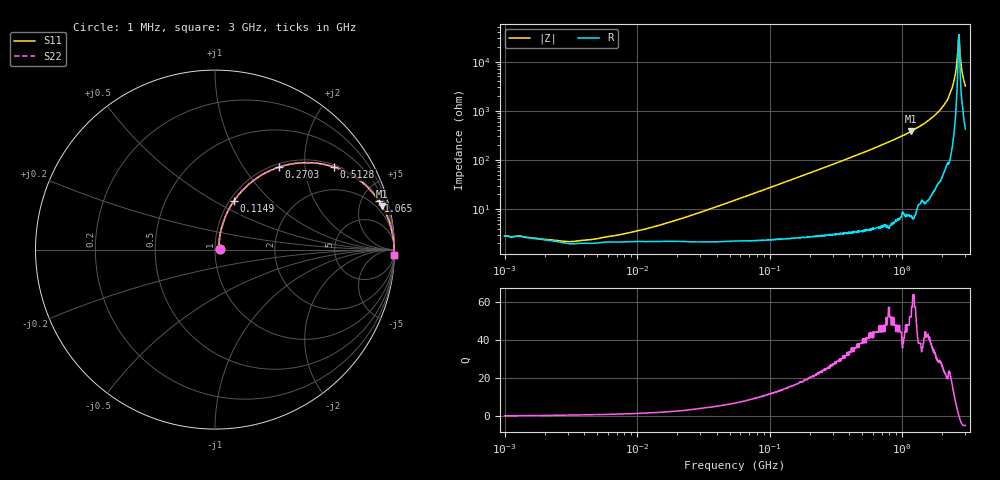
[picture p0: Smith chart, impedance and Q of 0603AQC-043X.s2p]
!s-Parameter Generated by FASTRON Sdn. Bhd.
!FASTRON P/N : 0603AQC-043X
!Keysight Technologies: E4991B_MY54100416_A.01.15
!Date: Thu Jun 25 13:54:13 2026
!Version  :Rev00  Thu Jun 25 13:54:13 2026
!Data & Calibration Information:
!Freq  S11  S21  S12  S22
!PortZ  Port1:50+j0  Port2:50+j0
!When reading reference impedance value at option line is always used.
! Remarks : This data is being provided solely for informational purposes.
# Hz S dB R 50
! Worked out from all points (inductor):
!   1601 points, 1 MHz to 3 GHz, reference 50 ohm
!   read as one part in series: L = 44 nH near 23.51 MHz
!   highest Q = 52.2 at 1.171 GHz (marker M1), where L = 52.1 nH
!   self-resonance near 2.674 GHz
!   S11 on the Smith chart (normalised r, x): 1 MHz: 1.06, +0.01; 114.9 MHz: 1.05, +0.62; 270.3 MHz: 1.06, +1.46; 512.8 MHz: 1.07, +2.84; 1.065 GHz: 1.14, +6.66; 3 GHz: 9, -63
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1000000  -31.30 5.8  -0.24 -0.2  -0.24 -0.2  -31.30 5.8
2961997  -33.40 22.9  -0.17 -0.5  -0.17 -0.5  -33.40 22.9
3804036  -33.00 28.3  -0.17 -0.6  -0.17 -0.6  -33.00 28.3
1.447069e7  -26.90 59.6  -0.19 -2.3  -0.19 -2.3  -26.90 59.6
5.504702e7  -16.60 73.2  -0.28 -8.4  -0.28 -8.4  -16.60 73.2
1.148668e8  -10.70 68.7  -0.59 -16.9  -0.59 -16.9  -10.70 68.7
2.083556e8  -6.36 58.5  -1.37 -28.7  -1.37 -28.7  -6.36 58.5
2.702786e8  -4.74 52.3  -2.02 -35.4  -2.02 -35.4  -4.74 52.3
5.128394e8  -1.85 34.7  -4.89 -53.8  -4.89 -53.8  -1.85 34.7
7.925923e8  -0.80 23.3  -8.07 -65.7  -8.07 -65.7  -0.80 23.3
1.064802e9  -0.42 16.6  -10.90 -72.2  -10.90 -72.2  -0.42 16.6
1.171007e9  -0.33 14.6  -12.00 -74.3  -12.00 -74.3  -0.33 14.6
1.712864e9  -0.11 7.5  -17.70 -80.9  -17.70 -80.9  -0.11 7.5
2.145442e9  -0.05 3.8  -23.70 -83.5  -23.70 -83.5  -0.05 3.8
2.289646e9  -0.03 2.6  -26.90 -84.9  -26.90 -84.9  -0.03 2.6
2.431346e9  -0.02 1.6  -31.10 -84.2  -31.10 -84.2  -0.02 1.6
2.51802e9  -0.02 1.0  -34.90 -81.8  -34.90 -81.8  -0.02 1.0
2.607784e9  -0.02 0.4  -41.90 -71.8  -41.90 -71.8  -0.02 0.4
2.660507e9  -0.02 0.1  -49.40 -37.7  -49.40 -37.7  -0.02 0.1
2.741597e9  -0.03 -0.4  -43.10 65.5  -43.10 65.5  -0.03 -0.4
2.882277e9  -0.04 -1.2  -33.70 77.5  -33.70 77.5  -0.04 -1.2
3e9  -0.04 -1.8  -30.10 80.6  -30.10 80.6  -0.04 -1.8
